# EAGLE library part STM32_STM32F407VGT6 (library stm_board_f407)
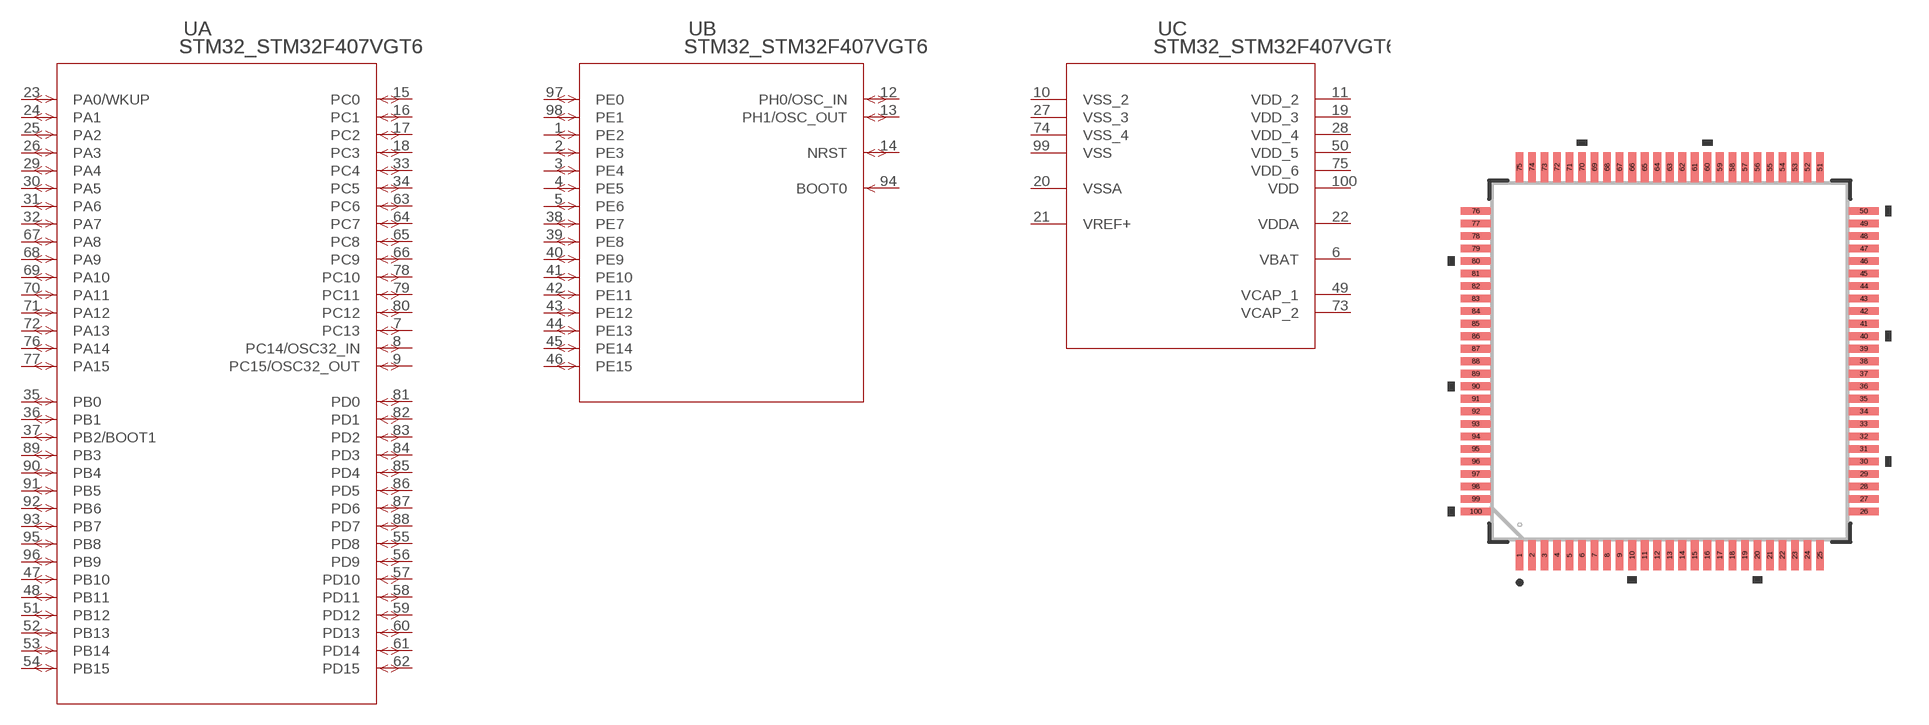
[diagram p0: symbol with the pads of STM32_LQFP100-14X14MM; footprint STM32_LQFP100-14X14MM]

Designator prefix U; gates A=STM32_STM32F4XXV2_1 B=STM32_STM32F4XXV2 C=STM32_STM32F4XXV2_00

## STM32_STM32F407VGT6 (BUILT_BY: EMA_UL_Team; COPYRIGHT: Copyright (C) 2018 Accelerated Designs. All rights reserved; MANUFACTURER_PART_NUMBER: STM32F407VGT6; SOURCELIBRARY: Updates_to_database_2020-10-19; VENDOR: STMicroelectronics)  [STM32_LQFP100-14X14MM]
1  B:PE2
2  B:PE3
3  B:PE4
4  B:PE5
5  B:PE6
6  C:VBAT  pwr
7  A:PC13
8  A:PC14/OSC32_IN
9  A:PC15/OSC32_OUT
10  C:VSS_2  pwr
11  C:VDD_2  pwr
12  B:PH0/OSC_IN
13  B:PH1/OSC_OUT
14  B:NRST
15  A:PC0
16  A:PC1
17  A:PC2
18  A:PC3
19  C:VDD_3  pwr
20  C:VSSA  pwr
21  C:VREF+  pwr
22  C:VDDA  pwr
23  A:PA0/WKUP
24  A:PA1
25  A:PA2
26  A:PA3
27  C:VSS_3  pwr
28  C:VDD_4  pwr
29  A:PA4
30  A:PA5
31  A:PA6
32  A:PA7
33  A:PC4
34  A:PC5
35  A:PB0
36  A:PB1
37  A:PB2/BOOT1
38  B:PE7
39  B:PE8
40  B:PE9
41  B:PE10
42  B:PE11
43  B:PE12
44  B:PE13
45  B:PE14
46  B:PE15
47  A:PB10
48  A:PB11
49  C:VCAP_1  pwr
50  C:VDD_5  pwr
51  A:PB12
52  A:PB13
53  A:PB14
54  A:PB15
55  A:PD8
56  A:PD9
57  A:PD10
58  A:PD11
59  A:PD12
60  A:PD13
61  A:PD14
62  A:PD15
63  A:PC6
64  A:PC7
65  A:PC8
66  A:PC9
67  A:PA8
68  A:PA9
69  A:PA10
70  A:PA11
71  A:PA12
72  A:PA13
73  C:VCAP_2  pwr
74  C:VSS_4  pwr
75  C:VDD_6  pwr
76  A:PA14
77  A:PA15
78  A:PC10
79  A:PC11
80  A:PC12
81  A:PD0
82  A:PD1
83  A:PD2
84  A:PD3
85  A:PD4
86  A:PD5
87  A:PD6
88  A:PD7
89  A:PB3
90  A:PB4
91  A:PB5
92  A:PB6
93  A:PB7
94  B:BOOT0  in
95  A:PB8
96  A:PB9
97  B:PE0
98  B:PE1
99  C:VSS  pwr
100  C:VDD  pwr

## Footprint STM32_LQFP100-14X14MM (pad centres in mm)
smd 0.305 x 1.194: 1 -6,-7.75; 2 -5.5,-7.75; 3 -5,-7.75; 4 -4.5,-7.75; 5 -4,-7.75; 6 -3.5,-7.75; 7 -3,-7.75; 8 -2.5,-7.75; 9 -2,-7.75; 10 -1.5,-7.75; 11 -1,-7.75; 12 -0.5,-7.75; 13 0,-7.75; 14 0.5,-7.75; 15 1,-7.75; 16 1.5,-7.75; 17 2,-7.75; 18 2.5,-7.75; 19 3,-7.75; 20 3.5,-7.75; 21 4,-7.75; 22 4.5,-7.75; 23 5,-7.75; 24 5.5,-7.75; 25 6,-7.75; 51 6,7.75; 52 5.5,7.75; 53 5,7.75; 54 4.5,7.75; 55 4,7.75; 56 3.5,7.75; 57 3,7.75; 58 2.5,7.75; 59 2,7.75; 60 1.5,7.75; 61 1,7.75; 62 0.5,7.75; 63 0,7.75; 64 -0.5,7.75; 65 -1,7.75; 66 -1.5,7.75; 67 -2,7.75; 68 -2.5,7.75; 69 -3,7.75; 70 -3.5,7.75; 71 -4,7.75; 72 -4.5,7.75; 73 -5,7.75; 74 -5.5,7.75; 75 -6,7.75
smd 1.194 x 0.305: 26 7.75,-6; 27 7.75,-5.5; 28 7.75,-5; 29 7.75,-4.5; 30 7.75,-4; 31 7.75,-3.5; 32 7.75,-3; 33 7.75,-2.5; 34 7.75,-2; 35 7.75,-1.5; 36 7.75,-1; 37 7.75,-0.5; 38 7.75,0; 39 7.75,0.5; 40 7.75,1; 41 7.75,1.5; 42 7.75,2; 43 7.75,2.5; 44 7.75,3; 45 7.75,3.5; 46 7.75,4; 47 7.75,4.5; 48 7.75,5; 49 7.75,5.5; 50 7.75,6; 76 -7.75,6; 77 -7.75,5.5; 78 -7.75,5; 79 -7.75,4.5; 80 -7.75,4; 81 -7.75,3.5; 82 -7.75,3; 83 -7.75,2.5; 84 -7.75,2; 85 -7.75,1.5; 86 -7.75,1; 87 -7.75,0.5; 88 -7.75,0; 89 -7.75,-0.5; 90 -7.75,-1; 91 -7.75,-1.5; 92 -7.75,-2; 93 -7.75,-2.5; 94 -7.75,-3; 95 -7.75,-3.5; 96 -7.75,-4; 97 -7.75,-4.5; 98 -7.75,-5; 99 -7.75,-5.5; 100 -7.75,-6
